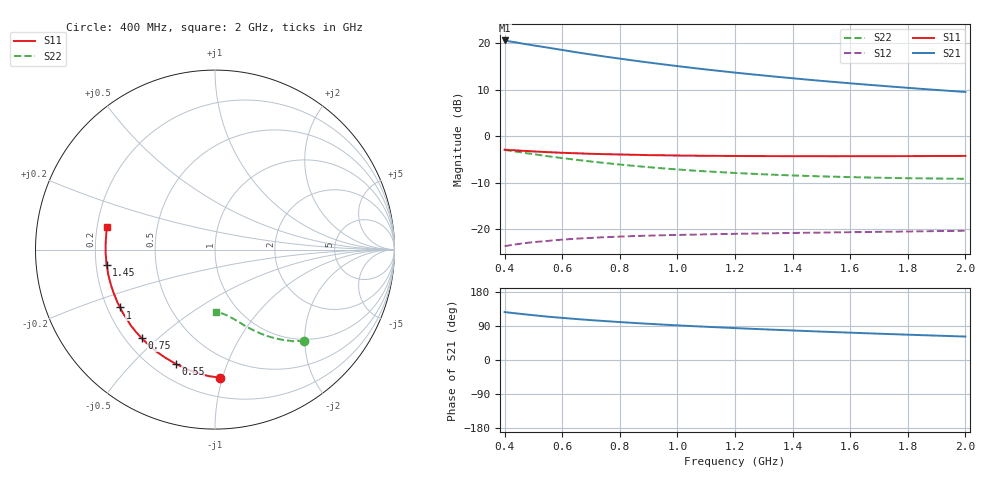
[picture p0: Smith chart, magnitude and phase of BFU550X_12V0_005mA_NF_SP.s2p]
! Filename:  P:\Prog\Test\Noise\ATS_data\Testdata_Net\BFU550X no attenuator noise\BFU550X_APG2013_44_C05_12p0V_005mA_NF_CM01_D.sf
! Date/Time: Fri 26/Jul/2013 14:37:14
! BFU550X_APG2013_44_C05_12p0V_1to10mA_NF_CM01_Bias4_R.sf
! Noise Parameter Data File
! BFU550X_APG2013_44_C05_12p0V_1to10mA_NF_CM01
! Date/time: Thu Jul 25 09:36:35 2013
! VAR V_out= 12.001000
! VAR I_out= 5.000000
! VAR V_in= 0.796800
! VAR I_in= 0.045405
! Device data file deembeded for feedlines and parallel
! Original file: \BFU550X no attenuator noise\BFU550X_APG2013_44_C05_12p0V_005mA_NF_CM01_R.sf
! Feed-files: PR005V01_100713_Feed1.s2p, PR005V01_100713_Feed2.s2p
! Parallel-file: PR005V01_100713_Par.s2p
# MHz S MA R 50
!  Freq-MHz  S11-mag  S11-arg  S21-mag  S21-arg  S12-mag  S12-arg  S22-mag  S22-arg
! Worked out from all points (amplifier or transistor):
!   37 points, 400 MHz to 2 GHz, reference 50 ohm
!   highest |S21| = 20.6 dB at 400 MHz (marker M1)
!   |S21| within 3 dB of that: start of sweep to 698.1 MHz
!   unconditionally stable (mu >= 1): nowhere
!   at 500 MHz: K = 0.26, MSG = 21.2 dB, |S12| = -22.8 dB
!   at 1.1 GHz: K = 0.54, MSG = 17.7 dB, |S12| = -21.1 dB
!   at 2 GHz: K = 0.88, MSG = 14.9 dB, |S12| = -20.3 dB
!   lowest NFmin = 0.67 dB at 440 MHz
!   S11 on the Smith chart (normalised r, x): 400 MHz: 0.34, -0.99; 550 MHz: 0.29, -0.67; 750 MHz: 0.26, -0.44; 1 GHz: 0.25, -0.26; 1.45 GHz: 0.24, -0.07; 2 GHz: 0.24, +0.10
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400  0.7156 -87.5  10.73 126.4  0.06551 47.3  0.7131 -45.7
420  0.7084 -90.6  10.45 124.7  0.06703 46.2  0.6959 -47.1
440  0.7037 -93.8  10.23 123.0  0.06861 45.0  0.6827 -48.3
460  0.697 -96.5  9.958 121.3  0.06994 43.9  0.6694 -49.7
500  0.6861 -102.2  9.501 118.2  0.07241 41.8  0.6423 -52.1
550  0.6734 -109.0  8.985 114.4  0.07466 39.6  0.6086 -54.8
600  0.6629 -114.7  8.479 111.1  0.07704 37.7  0.5816 -57.2
650  0.6551 -120.1  8 108.1  0.07895 36.1  0.557 -59.3
700  0.6467 -125.1  7.583 105.2  0.08044 34.7  0.5338 -61.3
750  0.6405 -129.6  7.186 102.6  0.08192 33.5  0.5143 -63.0
800  0.6357 -134.0  6.841 100.1  0.08311 32.4  0.4955 -64.8
850  0.6311 -138.1  6.513 97.8  0.08417 31.4  0.4791 -66.2
900  0.6257 -141.9  6.215 95.5  0.08504 30.6  0.4642 -67.6
950  0.6231 -145.4  5.939 93.4  0.08583 29.9  0.4507 -69.1
1000  0.6196 -148.7  5.682 91.4  0.08656 29.3  0.4388 -70.2
1100  0.6153 -154.7  5.227 87.7  0.08783 28.4  0.4183 -72.6
1200  0.6128 -160.2  4.84 84.2  0.08899 27.8  0.402 -74.7
1300  0.6109 -165.2  4.502 81.0  0.08998 27.3  0.389 -76.7
1450  0.6095 -172.0  4.07 76.4  0.09134 26.9  0.3738 -79.5
1500  0.6092 -174.1  3.941 74.9  0.09173 26.9  0.3695 -80.4
1750  0.6101 176.3  3.408 68.1  0.09382 27.1  0.3551 -84.6
2000  0.6141 168.0  2.996 61.9  0.09606 28.0  0.348 -88.6
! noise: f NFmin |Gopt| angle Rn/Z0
400  0.7182  0.1899  35.2  0.1201
460  0.6935  0.1355  62.21  0.0948
600  0.737  0.1628  67.08  0.1117
800  0.7619  0.1968  86.4  0.0953
1000  0.8114  0.2193  99.93  0.0915
1200  0.8502  0.2569  116.8  0.0828
1400  0.8762  0.2852  129.8  0.0768
1600  0.9216  0.3174  144.4  0.0616
1800  0.934  0.3503  156.7  0.0562
2000  0.9887  0.3828  169.8  0.0489
